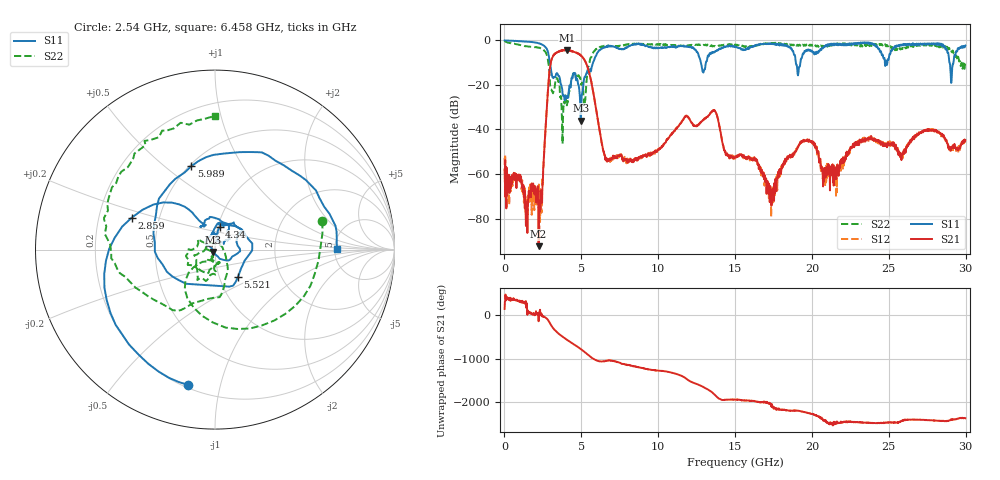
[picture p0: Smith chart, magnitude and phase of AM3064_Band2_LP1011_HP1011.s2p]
# Hz S DB R 50.0
!freq dBS11 angS11 dBS21 angS21 dBS12 angS12 dBS22 angS22
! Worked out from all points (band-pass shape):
!   1600 points, 10 MHz to 29.98 GHz, reference 50 ohm
!   highest |S21| = -4.40 dB at 4.077 GHz (marker M1); lowest = -92.4 dB at 2.222 GHz (marker M2)
!   |S21| within 3 dB of the highest: 3.142 GHz to 5.058 GHz (1.915 GHz wide, 46.7 % of centre)
!   lowest |S11| = -36.0 dB at 4.958 GHz (marker M3), VSWR 1.03, Z = 49.1 - j1.32 ohm
!   |S11| at or under -10 dB: 2.956 GHz to 5.758 GHz (2.801 GHz wide, 64.3 % of centre); 12.78 GHz to 13.1 GHz (320 MHz wide, 2.47 % of centre); 18.95 GHz to 19.25 GHz (297.8 MHz wide, 1.56 % of centre)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
!   |S22| runs from -46.5 to -0.3 dB; largest |S21 - S12| = 0.019
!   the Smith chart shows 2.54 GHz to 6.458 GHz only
!   S11 on the Smith chart (normalised r, x): 2.54 GHz: 0.22, -0.80; 2.859 GHz: 0.35, +0.16; 4.34 GHz: 1.02, +0.26; 5.521 GHz: 1.23, -0.39; 5.989 GHz: 0.51, +0.62; 6.458 GHz: 5.23, +0.07
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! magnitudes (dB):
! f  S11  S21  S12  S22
! 10 MHz  0.0  -58.1  -52.7  -0.3
! 2.222 GHz  -1.3  -92.4  -69.8  -3.3
! 2.54 GHz  -2.3  -56.8  -54.6  -4.2
! 2.859 GHz  -6.1  -19.5  -19.6  -10.1
! 3.178 GHz  -17.0  -6.9  -6.9  -23.3
! 4.077 GHz  -25.8  -4.4  -4.5  -28.6
! 4.34 GHz  -17.8  -4.9  -4.7  -18.2
! 4.958 GHz  -36.0  -6.8  -6.7  -17.9
! 5.015 GHz  -25.5  -7.1  -7.1  -20.0
! 5.521 GHz  -14.1  -14.7  -14.7  -10.5
! 5.989 GHz  -6.3  -32.3  -32.1  -3.9
! 6.458 GHz  -3.4  -50.4  -50.2  -2.5
! 10 GHz  -3.4  -49.2  -48.9  -1.9
! 13.6 GHz  -5.2  -31.7  -31.5  -2.5
! 15 GHz  -2.7  -52.5  -53.1  -1.9
! 17.44 GHz  -1.7  -67.1  -66.1  -1.5
! 19.99 GHz  -4.6  -45.9  -45.9  -1.9
! 20.82 GHz  -2.8  -61.9  -59.1  -2.3
! 25 GHz  -8.4  -46.5  -46.5  -2.3
! 28.28 GHz  -1.4  -41.3  -40.9  -3.1
! 29.08 GHz  -17.8  -48.1  -48.0  -5.1
! 29.98 GHz  -2.3  -44.9  -45.8  -10.3
